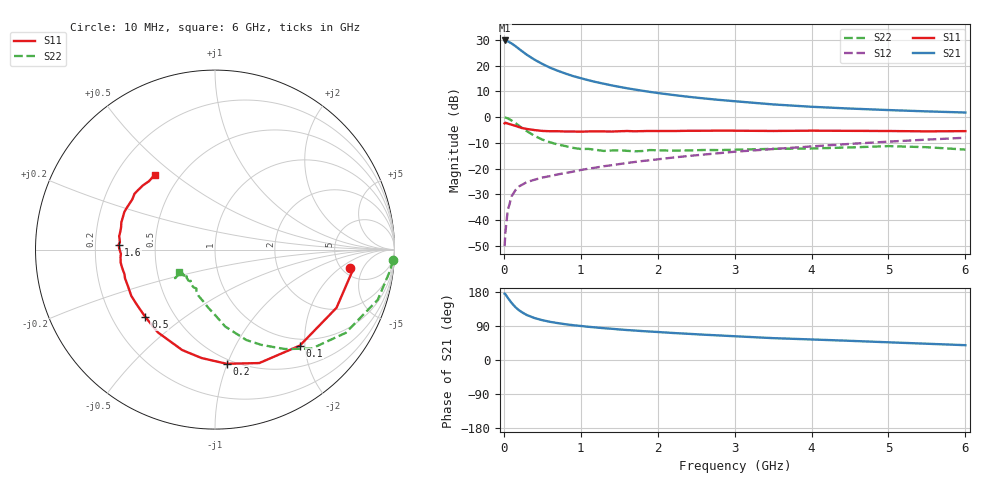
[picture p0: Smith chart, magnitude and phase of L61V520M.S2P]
!  INFINEON TECHNOLOGIES Small Signal Semiconductors
! BFR380L3 , Si-NPN RF-Transistor in TSLP-3-1
!  Vce=1.5 V,  Ic=20 mA
! Common Emitter S-Parameters:  07. March 2005
#  GHz  S  MA  R  50
! f  S11  S21  S12  S22
! GHz  Mag  Ang  Mag  Ang  Mag  Ang  Mag  Ang
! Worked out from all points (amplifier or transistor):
!   36 points, 10 MHz to 6 GHz, reference 50 ohm
!   highest |S21| = 29.8 dB at 10 MHz (marker M1)
!   |S21| within 3 dB of that: start of sweep to 185.1 MHz
!   unconditionally stable (mu >= 1): 1.93 GHz to 4.933 GHz
!   at 250 MHz: K = 0.35, MSG = 25.7 dB, |S12| = -26.1 dB
!   at 1.4 GHz: K = 0.95, MSG = 15.5 dB, |S12| = -18.7 dB
!   at 6 GHz: K = 0.98, MSG = 4.9 dB, |S12| = -8.0 dB
!   S11 on the Smith chart (normalised r, x): 10 MHz: 5.89, -2.81; 100 MHz: 0.87, -1.90; 200 MHz: 0.46, -0.99; 500 MHz: 0.34, -0.36; 1.6 GHz: 0.30, +0.02; 6 GHz: 0.36, +0.43
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0.01  0.7581 -7.7  31.02 175.0  0.0031 85.6  0.9948 -3.4
0.02  0.7795 -7.6  30.68 173.9  0.0057 87.1  0.9813 -7.1
0.05  0.7506 -25.6  29.92 164.4  0.015 79.4  0.9491 -17.1
0.1  0.7139 -48.5  27.18 150.9  0.0287 68.8  0.8635 -32.5
0.15  0.6785 -68.7  24.13 139.5  0.038 60.7  0.7705 -45.7
0.2  0.6394 -84.2  21.09 130.8  0.0452 56.2  0.6771 -54.9
0.25  0.6087 -97.1  18.54 124.2  0.0497 52.7  0.5915 -63.9
0.3  0.5887 -108.1  16.31 118.6  0.0548 50.9  0.5341 -70.8
0.4  0.5605 -124.6  13.09 110.6  0.0608 49.3  0.4319 -82.5
0.5  0.5402 -135.9  10.85 105.1  0.0669 49.4  0.3667 -89.6
0.6  0.5328 -144.6  9.177 100.7  0.0714 49.8  0.3256 -96.7
0.8  0.526 -157.2  7.057 94.4  0.082 52.5  0.2741 -109.4
0.9  0.5262 -162.2  6.297 91.9  0.0872 53.4  0.2529 -114.0
1.1  0.5274 -169.0  5.224 87.6  0.0995 55.5  0.2414 -120.3
1.3  0.5281 -175.4  4.468 83.9  0.1111 57.2  0.2204 -128.0
1.6  0.5381 177.2  3.652 79.1  0.1283 58.7  0.2216 -135.9
2.2  0.5375 166.9  2.702 71.3  0.1638 60.7  0.2236 -139.6
2.8  0.5467 157.6  2.167 64.8  0.1995 61.5  0.229 -145.8
3.5  0.5391 148.8  1.77 57.7  0.2398 60.2  0.242 -145.3
4.5  0.542 142.4  1.47 50.6  0.3022 59.3  0.2579 -145.0
5.5  0.5297 134.0  1.295 42.9  0.3661 55.8  0.2605 -145.2
6  0.535 128.8  1.231 39.1  0.3982 53.8  0.2341 -148.3
